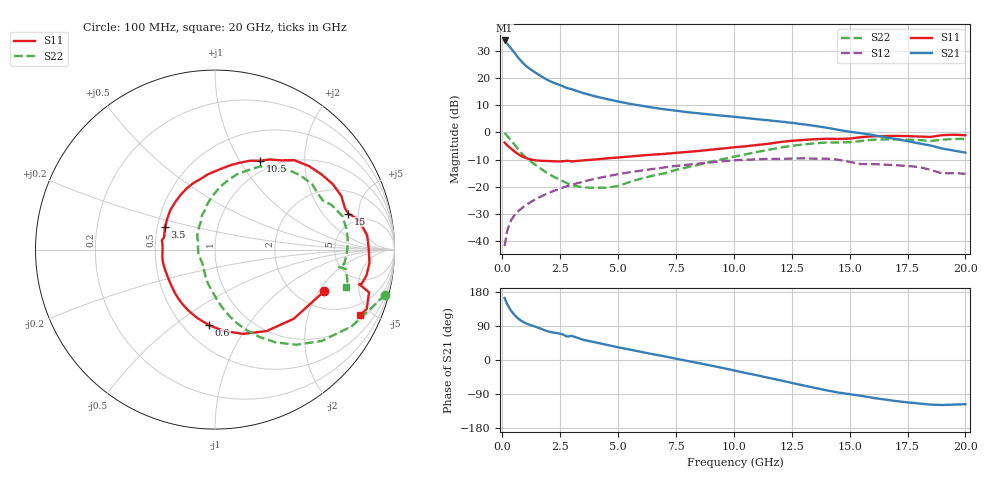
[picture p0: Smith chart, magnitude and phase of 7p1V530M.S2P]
! Infineon Technologies  Discrete & RF Semiconductors
! bfp620
! VCE =  1.5 V,  IC =  30 mA
! Common Emitter S-Parameters:  Sep 2002
# GHz  S  MA  R  50
!  f  S11  S21  S12  S22
! GHz  MAG  ANG  MAG  ANG  MAG  ANG  MAG  ANG
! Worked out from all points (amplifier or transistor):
!   59 points, 100 MHz to 20 GHz, reference 50 ohm
!   highest |S21| = 33.9 dB at 100 MHz (marker M1)
!   |S21| within 3 dB of that: start of sweep to 383.7 MHz
!   unconditionally stable (mu >= 1): 3.119 GHz to 9.871 GHz; 17.18 GHz to end of sweep
!   at 1 GHz: K = 0.77, MSG = 25.8 dB, |S12| = -26.9 dB
!   at 5.5 GHz: K = 1.04, MAG = 11.5 dB, |S12| = -14.7 dB
!   at 20 GHz: K = 1.32, MAG = 0.5 dB, |S12| = -15.2 dB
!   S11 on the Smith chart (normalised r, x): 100 MHz: 2.78, -2.24; 600 MHz: 0.66, -0.68; 3.5 GHz: 0.55, +0.15; 10.5 GHz: 0.86, +1.23; 15 GHz: 3.84, +3.76; 20 GHz: 1.24, -4.30
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0.1  0.6512 -20.9  49.65 163.6  0.008 84.0  0.9809 -14.9
0.2  0.5839 -41.3  43.69 149.0  0.0147 73.3  0.8733 -29.3
0.3  0.5372 -57.7  38.87 137.5  0.0202 68.4  0.7832 -40.5
0.4  0.4952 -71.5  34.47 128.3  0.0248 65.2  0.6982 -49.4
0.5  0.4563 -83.6  30.4 120.7  0.0287 62.9  0.6181 -56.8
0.6  0.4224 -94.5  26.76 114.3  0.0323 61.4  0.5455 -63.1
0.7  0.3944 -104.3  23.63 108.8  0.0356 60.3  0.4825 -68.5
0.8  0.3721 -113.0  21.03 104.2  0.0388 59.5  0.4296 -73.2
0.9  0.3546 -120.5  18.92 100.4  0.0419 59.0  0.3861 -77.1
1.1  0.3294 -132.5  15.86 94.7  0.048 58.3  0.322 -83.2
1.3  0.3132 -142.0  13.78 90.5  0.0543 57.7  0.2768 -87.9
2  0.2974 -169.4  9.061 75.0  0.0765 54.3  0.172 -106.6
2.8  0.3009 170.0  6.568 61.9  0.1022 48.7  0.1154 -128.6
3  0.292 166.1  6.255 63.6  0.1084 47.0  0.1065 -129.1
3.5  0.3055 156.0  5.305 53.3  0.1244 42.7  0.0965 -146.9
5  0.3451 130.0  3.719 33.6  0.1699 28.8  0.1028 156.2
7  0.4021 101.3  2.675 9.7  0.2267 9.6  0.176 116.3
10.5  0.5546 63.2  1.848 -34.1  0.3139 -29.8  0.3937 79.2
13.5  0.7508 29.1  1.319 -73.5  0.3299 -65.9  0.6302 41.2
15  0.7689 15.1  1.031 -90.1  0.286 -87.0  0.6606 24.4
17  0.8637 -5.0  0.756 -108.3  0.2484 -97.5  0.7414 2.8
20  0.888 -24.3  0.425 -116.5  0.1731 -107.6  0.7598 -15.8
